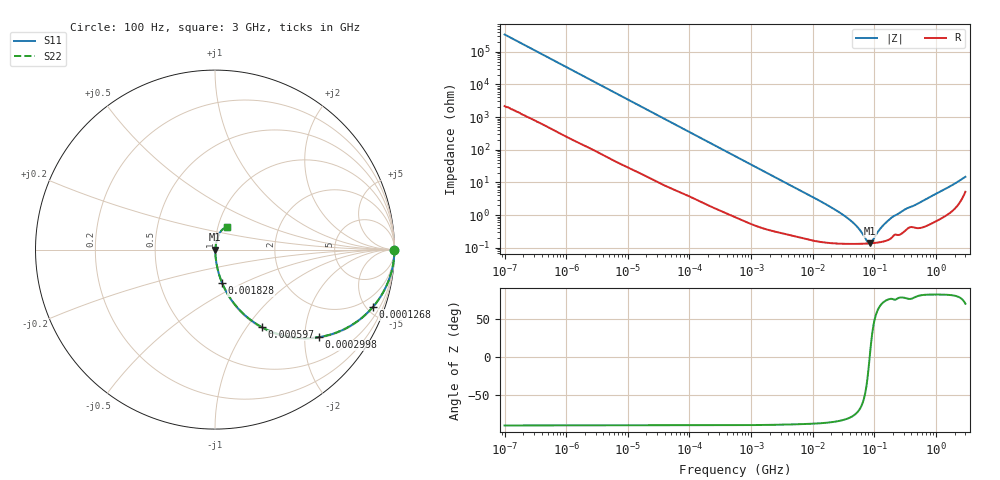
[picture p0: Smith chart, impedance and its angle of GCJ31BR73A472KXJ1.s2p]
!Murata Part Number: GCJ31BR73A472KXJ1
!These Parameters are Measured in Series Mode Connection
!Data Generated on Mar 13, 2026
!  o--ll--o
!Port1  Port2
!  o------o
!Operation Temp=25[degC], DC Bias Voltage=0[V]
!Freq. Start=100[Hz] Stop=3[GHz] 401[Steps]
# Hz S RI R 50
!Freq.(Hz) S11(Real) S11(Imag) S21(Real) S21(Imag) S12(Real) S12(Imag) S22(Real) S22(Imag)
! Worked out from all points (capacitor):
!   401 points, 100 Hz to 3 GHz, reference 50 ohm
!   read as one part in series: C = 4.72 nF near 109 Hz
!   lowest |Z| = 137 mohm at 84.26 MHz (marker M1)
!   series resonance near 83.95 MHz, so ESL is about 760 pH
!   S11 on the Smith chart (normalised r, x): 100 Hz: open; 126.8 kHz: 1.06, -5.51; 299.8 kHz: 1.03, -2.34; 597 kHz: 1.02, -1.18; 1.828 MHz: 1.01, -0.39; 3 GHz: 1.10, +0.28
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100  1 -0.000297  2e-06 0.000297  2e-06 0.000297  1 -0.000297
1788  0.9999 -0.00524  6.77e-05 0.00524  6.77e-05 0.00524  0.9999 -0.00524
31977  0.9907 -0.0914  0.00926 0.0914  0.00926 0.0914  0.9907 -0.0914
72443  0.9566 -0.1988  0.0434 0.1988  0.0434 0.1988  0.9566 -0.1988
126767  0.8809 -0.3184  0.1191 0.3184  0.1191 0.3184  0.8809 -0.3184
194955  0.761 -0.4208  0.239 0.4208  0.239 0.4208  0.761 -0.4208
299821  0.5777 -0.4879  0.4223 0.4879  0.4223 0.4879  0.5777 -0.4879
547723  0.2959 -0.4497  0.7041 0.4497  0.7041 0.4497  0.2959 -0.4497
596961  0.2621 -0.433  0.7379 0.433  0.7379 0.433  0.2621 -0.433
1000599  0.1151 -0.3118  0.8849 0.3118  0.8849 0.3118  0.1151 -0.3118
1827928  0.0397 -0.1862  0.9603 0.1862  0.9603 0.1862  0.0397 -0.1862
9794414  0.00299 -0.0363  0.997 0.0363  0.997 0.0363  0.00299 -0.0363
2.316512e7  0.00157 -0.0145  0.9984 0.0145  0.9984 0.0145  0.00157 -0.0145
3.882828e7  0.00137 -0.00735  0.9986 0.00735  0.9986 0.00735  0.00137 -0.00735
5.248048e7  0.00133 -0.00422  0.9987 0.00422  0.9987 0.00422  0.00133 -0.00422
7.730952e7  0.00135 -0.000714  0.9987 0.000714  0.9987 0.000714  0.00135 -0.000714
8.425944e7  0.00136 3.28e-05  0.9986 -3.28e-05  0.9986 -3.28e-05  0.00136 3.28e-05
9.183415e7  0.00138 0.000781  0.9986 -0.000781  0.9986 -0.000781  0.00138 0.000781
1.295826e8  0.00152 0.00391  0.9985 -0.00391  0.9985 -0.00391  0.00152 0.00391
1.751444e8  0.00185 0.00708  0.9982 -0.00708  0.9982 -0.00708  0.00185 0.00708
3.199599e8  0.0036 0.0148  0.9964 -0.0148  0.9964 -0.0148  0.0036 0.0148
3e9  0.0655 0.124  0.9345 -0.124  0.9345 -0.124  0.0655 0.124
